|Texas Instruments Incorporated
|Octal Low power 12-bit +/-15V Output Serial Input Digital-to-Analog Converter
| Marketing part#   Digital Voltage Range   Package-type   #pins
| DAC7718SPAG   1.8 - 5.5V   TQFP   64
| DAC7718SPAGR   1.8 - 5.5V   TQFP   64
| DAC7718SRGZR   1.8 - 5.5V   VQFN   48
| DAC7718SRGZT   1.8 - 5.5V   VQFN   48
[IBIS Ver]   3.2
[File name]   dac7718.ibs
|SIMDE Ver   V2.2 - 201009 - RHL4 - Build 424
[File Rev]   1.0
[Date]   01/11/2011
[Source]
| Texas Instruments Incorporated.
| Analog-eLab Design Center, HPA
| 12500 TI Blvd
| Dallas, TX -75243
| e-mail: elab_ibis@list.ti.com
| -Model generated from simulations in TISPICE
[Notes]   Revision History:
| Rev 1.0: 01/11/2011
| - Initial version of the model
| - Model generated from simulations in TISPICE
| - Model matched to SPICE simulation
| - C_comp although listed in numerical order of value are
|   obtained from varying PVT conditions. For PVT conditions for
|   each specific value refer the buffer description under
|   respective [Model]. IBIS model user is responsible for using
|   appropriate C_comp to simulate for Signal Integrity.
| - Model names with a trailing _2 contains the model for
|   2V [1.8V and 2.2V].Model names with a trailing _3p3 contains
|   the model for 3.3V [3.0V and 3.6V]. Model names with trailing _5
|   contains the model for 5.0V [4.5V and 5.5V] operation.
[Disclaimer]
| This model is designed as an aid for customers of Texas Instruments.
| TI and its licensors and suppliers make no warranties, either expressed
| or implied, with respect to this  model, including the warranties of
| merchantability or fitness for a particular purpose. The model is
| provided solely on an "as is" basis. The entire risk as to its quality
| and performance is with the customer.
[Copyright]
 (C) Copyright 2011 Texas Instruments Incorporated.All rights reserved.
|   DAC7718PAG
[Component]   DAC7718PAG
[Manufacturer]   TI
[Package]   |64 TQFP  -  PAG package
|   typ   min   max
R_pkg   0.09662   0.05590   0.10573
L_pkg   3.25825nH   2.87218nH   3.41861nH
C_pkg   0.50100pF   0.43676pF   0.52522pF
[Pin]  signal_name   model_name   R_pin   L_pin   C_pin
1   Avdd   POWER   0.05853   3.25275nH  0.49570pF
2   NC   NC   0.00979   2.07533nH  0.44422pF
3   AIN-0   TERM   0.09916   3.34220nH  0.52255pF
4   VOUT-3   TERM   0.10572   3.41858nH  0.51361pF
5   REF-A   TERM   0.10298   3.34083nH  0.50499pF
6   VOUT-2   TERM   0.10520   3.32054nH  0.48841pF
7   VOUT-1   TERM   0.10315   3.22810nH  0.47964pF
8   AGND-A   GND   0.05617   2.87447nH  0.48185pF
9   AGND-A   GND   0.05633   2.88143nH  0.48269pF
10   OFFSET-A   TERM   0.05590   2.87229nH  0.51348pF
11   VOUT-0   TERM   0.10169   3.25862nH  0.48167pF
12   AVSS   POWER   0.05522   2.97650nH  0.52803pF
13   NC   NC   0.00937   1.95351nH  0.41976pF
14   VMON   TERM   0.09903   3.33957nH  0.51710pF
15   NC   NC   0.00979   2.07450nH  0.44472pF
16   NC   NC   0.00987   2.17284nH  0.36892pF
17   NC   NC   0.00987   2.17294nH  0.36893pF
18   NC   NC   0.00979   2.07533nH  0.44422pF
19   GPIO-2   GPIO   0.09490   3.26989nH  0.51566pF
20   _CLR   INPUT_ISO   0.09650   3.25657nH  0.50208pF
21   _RST   INPUT_ISO   0.09693   3.23623nH  0.49298pF
22   NC   NC   0.00916   1.86104nH  0.39171pF
23   NC   NC   0.00889   1.80020nH  0.38069pF
24   DVDD   POWER   0.05373   2.72080nH  0.46920pF
25   DGND   GND   0.05386   2.70392nH  0.47141pF
26   NC   NC   0.00889   1.80025nH  0.38065pF
27   NC   NC   0.00917   1.86172nH  0.39156pF
28   DGND   GND   0.09628   3.22448nH  0.49134pF
29   GPIO-1   GPIO   0.09531   3.23498nH  0.50141pF
30   GPIO-0   GPIO   0.09459   3.26362nH  0.51697pF
31   NC   NC   0.00979   2.07445nH  0.44475pF
32   NC   NC   0.00986   2.17258nH  0.36899pF
33   NC   NC   0.00987   2.17293nH  0.36893pF
34   NC   NC   0.00979   2.07533nH  0.44422pF
35   NC   NC   0.00952   1.99850nH  0.43874pF
36   NC   NC   0.00937   1.95358nH  0.41947pF
37   AVSS   POWER   0.05522   2.97543nH  0.52636pF
38   VOUT-7   TERM   0.10169   3.25804nH  0.48176pF
39   OFFSET-B   TERM   0.05591   2.87218nH  0.51349pF
40   AGND-B   GND   0.05633   2.87986nH  0.48278pF
41   AGND-B   GND   0.05618   2.87609nH  0.48176pF
42   VOUT-6   TERM   0.10316   3.22827nH  0.47960pF
43   VOUT-5   TERM   0.10521   3.32132nH  0.48826pF
44   REF-B   TERM   0.10299   3.34109nH  0.50503pF
45   VOUT-4   TERM   0.10573   3.41861nH  0.51389pF
46   AIN-1   TERM   0.09916   3.34187nH  0.52310pF
47   NC   NC   0.00979   2.07450nH  0.44472pF
48   AVdd   POWER   0.05853   3.25559nH  0.49503pF
49   NC   NC   0.00987   2.17295nH  0.36893pF
50   _USB/BTC   INPUT   0.09804   3.38993nH  0.52489pF
51   RSTSEL   INPUT   0.09893   3.33419nH  0.52031pF
52   NC   NC   0.00936   1.95355nH  0.41948pF
53   NC   NC   0.00943   1.92643nH  0.41193pF
54   DGND   GND   0.05428   2.78415nH  0.52065pF
55   IOVDD   POWER   0.09848   3.13890nH  0.47475pF
56   DVDD   POWER   0.05463   2.68397nH  0.49140pF
57   SCLK   INPUT_ISO   0.09978   3.15860nH  0.43676pF
58   _CS   INPUT_ISO   0.09830   3.13575nH  0.46977pF
59   SDI   INPUT_ISO   0.09748   3.17722nH  0.47289pF
60   NC   NC   0.00943   1.92658nH  0.41197pF
61   SDO   SDO   0.09630   3.24398nH  0.50026pF
62   _LDAC   INPUT_ISO   0.09572   3.27512nH  0.52224pF
63   _WAKEUP   INPUT_ISO   0.09604   3.35275nH  0.52522pF
64   NC   NC   0.00986   2.17258nH  0.36899pF
|   DAC7718RGZ
[Component]   DAC7718RGZ
[Manufacturer]   TI
[Package]   |48 VQFN  -  RGZ package
|   typ   min   max
R_pkg   0.04181   0.02478   0.05004
L_pkg   1.03794nH   0.90966nH   1.23377nH
C_pkg   0.15178pF   0.13764pF   0.20084pF
[Pin]  signal_name   model_name   R_pin   L_pin   C_pin
1   Avdd   POWER   0.02261   0.79459nH  0.17672pF
2   AIN-0   TERM   0.04128   1.00362nH  0.14794pF
3   Vout-3   TERM   0.04504   1.10077nH  0.15413pF
4   REF-A   TERM   0.04087   0.99199nH  0.14703pF
5   Vout-2   TERM   0.04069   0.98748nH  0.14682pF
6   Vout-1   TERM   0.04126   1.00216nH  0.15065pF
7   AGND-A   GND   0.02230   0.78764nH  0.19167pF
8   AGND-A   GND   0.02365   0.85486nH  0.20048pF
9   OFFSET-A   TERM   0.02478   0.91014nH  0.20084pF
10   Vout-0   TERM   0.05004   1.23377nH  0.16625pF
11   Avss   POWER   0.02612   0.99974nH  0.19492pF
12   Vmon   TERM   0.04439   1.08949nH  0.13764pF
13   GPIO-2   GPIO   0.04795   1.18388nH  0.14501pF
14   _CLR   INPUT_ISO   0.04729   1.16131nH  0.15836pF
15   _RST   INPUT_ISO   0.04339   1.05637nH  0.14938pF
16   NC   NC   0.00077   0.11662nH  0.07856pF
17   DVdd   POWER   0.02070   0.66574nH  0.17579pF
18   NC   NC   0.00077   0.11658nH  0.07856pF
19   NC   NC   0.00077   0.11658nH  0.07856pF
20   DGND   GND   0.02110   0.67405nH  0.17897pF
21   NC   NC   0.00077   0.11663nH  0.07856pF
22   DGND   GND   0.04168   1.00478nH  0.14479pF
23   GPIO-1   GPIO   0.04381   1.06073nH  0.15121pF
24   GPIO-0   GPIO   0.04703   1.15038nH  0.14307pF
25   NC   NC   0.00077   0.12248nH  0.06703pF
26   AVss   POWER   0.02612   0.99589nH  0.19248pF
27   Vout-7   TERM   0.05004   1.22567nH  0.16593pF
28   OFFSET-B   TERM   0.02478   0.90966nH  0.20049pF
29   AGND-B   GND   0.02366   0.85298nH  0.20007pF
30   AGND-B   GND   0.02230   0.78471nH  0.19123pF
31   Vout-6   TERM   0.04127   0.99162nH  0.15023pF
32   Vout-5   TERM   0.04070   0.97669nH  0.14641pF
33   REF-B   TERM   0.04087   0.98131nH  0.14662pF
34   Vout-4   TERM   0.04504   1.09152nH  0.15379pF
35   AIN-1   TERM   0.04129   0.99309nH  0.14753pF
36   AVdd   POWER   0.02261   0.78596nH  0.17560pF
37   _USB/BTC   INPUT   0.04555   1.11142nH  0.14143pF
38   RSTSEL   INPUT   0.04360   1.05535nH  0.14859pF
39   NC   NC   0.00077   0.11677nH  0.07855pF
40   DGND   GND   0.02074   0.66234nH  0.18123pF
41   IOVdd   POWER   0.03904   0.93803nH  0.14577pF
42   DVdd   POWER   0.01991   0.60436nH  0.18642pF
43   SCLK   INPUT_ISO   0.03915   0.94075nH  0.14385pF
44   _CS   INPUT_ISO   0.03874   0.93316nH  0.14253pF
45   SDI   INPUT_ISO   0.03956   0.95500nH  0.14124pF
46   SDO   SDO   0.03879   0.93461nH  0.14010pF
47   _LDAC   INPUT_ISO   0.04021   0.97287nH  0.14445pF
48   _WAKEUP   INPUT_ISO   0.04322   1.05762nH  0.13839pF
|   Model Selectors
[Model Selector] INPUT_ISO
input_iso_2   2.0V digital input
input_iso_3p3  3.3V digital input
input_iso_5   5.0V digital input
[Model Selector] SDO
sdo_2   2.0V 3-state output
sdo_3p3   3.3V 3-state output
sdo_5   5.0V 3-state output
[Model Selector] INPUT
input_2   2.0V digital input
input_3p3   3.3V digital input
input_5   5.0V digital input
[Model Selector] GPIO
gpio_2   2.0V digital I/O_open_drain
gpio_3p3   3.3V digital I/O_open_drain
gpio_5   5.0V digital I/O_open_drain
[Model Selector] TERM
term_2-0V  2.0V nominal termination
term_3-3V  3.3V nominal termination
term_5-0V  5.0V nominal termination
[Model]  term_2-0V
Model_type Terminator
C_comp   1.0e-20F  1.0e-20F  1.0e-20F
|   typ   min   max
[Voltage Range]   2.0V   1.8V   2.2V
[POWER Clamp Reference]   2.0V   1.8V   2.2V
[GND Clamp Reference]   0V   0V   0V
|Ambient Temperature   25   85   -40
|Junction Temperature
[Temperature Range]   33   113   -40
[Model]  term_3-3V
Model_type Terminator
C_comp   1.0e-20F  1.0e-20F  1.0e-20F
|   typ   min   max
[Voltage Range]   3.3V   3.0V   3.6V
[POWER Clamp Reference]   3.3V   3.0V   3.6V
[GND Clamp Reference]   0V   0V   0V
|Ambient Temperature   25   85   -40
|Junction Temperature
[Temperature Range]   33   113   -40
[Model]  term_5-0V
Model_type Terminator
C_comp   1.0e-20F  1.0e-20F  1.0e-20F
|   typ   min   max
[Voltage Range]   5.0V   4.5V   5.5V
[POWER Clamp Reference]   5.0V   4.5V   5.5V
[GND Clamp Reference]   0V   0V   0V
|Ambient Temperature   25   85   -40
|Junction Temperature
[Temperature Range]   33   113   -40
| Models and submodels in the file (15): input_iso_2 (Input), input_iso_3p3 (Input), input_iso_5 (Input), sdo_2 (3-state), sdo_3p3 (3-state), sdo_5 (3-state), input_2 (Input), input_3p3 (Input), input_5 (Input), gpio_2 (I/O_open_drain), gpio_3p3 (I/O_open_drain), gpio_5 (I/O_open_drain), term_2-0V (Terminator), term_3-3V (Terminator), term_5-0V (Terminator)
